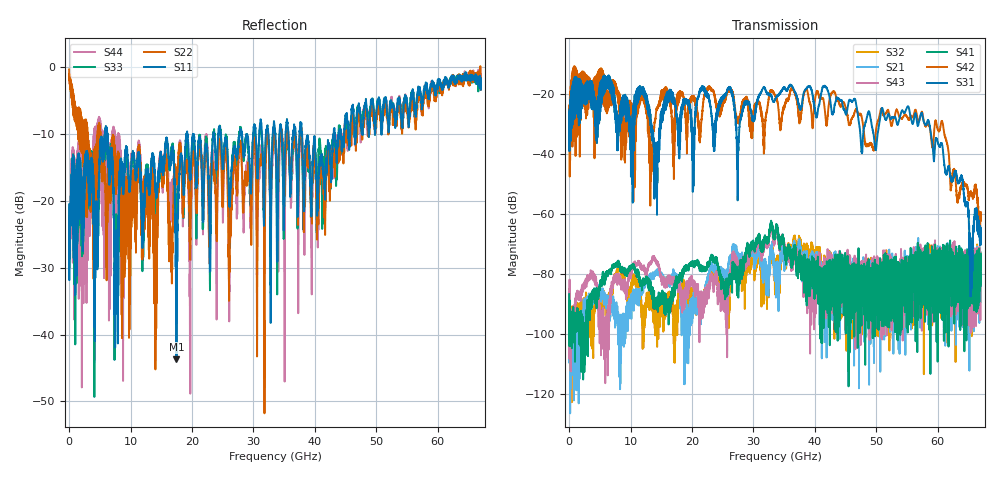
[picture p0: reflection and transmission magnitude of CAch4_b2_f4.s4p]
!Agilent Technologies,N5247A,US51170199,A.09.90.13
!Agilent N5247A: A.09.90.13
!Date: Thursday, October 18, 2018 11:44:51
!Correction: S11(Full 4 Port(1,2,3,4))
!S12(Full 4 Port(1,2,3,4))
!S13(Full 4 Port(1,2,3,4))
!S14(Full 4 Port(1,2,3,4))
!S21(Full 4 Port(1,2,3,4))
!S22(Full 4 Port(1,2,3,4))
!S23(Full 4 Port(1,2,3,4))
!S24(Full 4 Port(1,2,3,4))
!S31(Full 4 Port(1,2,3,4))
!S32(Full 4 Port(1,2,3,4))
!S33(Full 4 Port(1,2,3,4))
!S34(Full 4 Port(1,2,3,4))
!S41(Full 4 Port(1,2,3,4))
!S42(Full 4 Port(1,2,3,4))
!S43(Full 4 Port(1,2,3,4))
!S44(Full 4 Port(1,2,3,4))
!S4P File: Measurements: <S11,S12,S13,S14>,
!<S21,S22,S23,S24>,
!<S31,S32,S33,S34>,
!<S41,S42,S43,S44>:
# Hz S  dB  R 50
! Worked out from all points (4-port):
!   6701 points, 10 MHz to 67 GHz, reference 50 ohm
!   strongest paths, dB at 10 MHz, 16.76 GHz, 33.51 GHz, 50.25 GHz, 67 GHz:
!     S31: -30.8, -22.6, -21.9, -32.7, -65.4
!     S42: -29.6, -28.7, -20.3, -28.8, -59.4
!     S41: -86.7, -85.6, -66.7, -78.8, -83.8
!     S43: -85.9, -82.6, -67.4, -80.2, -76.8
!     S21: -85.4, -80.2, -81.8, -79.9, -77.8
!     S32: -91.4, -88.6, -79.1, -93.8, -72.9
!   lowest |S11| = -43.7 dB at 17.48 GHz (marker M1), VSWR 1.01, Z = 49.3 - j0.0152 ohm
!   |S11| at or under -10 dB: start of sweep to 5.848 GHz; 6.251 GHz to 19.13 GHz (12.88 GHz wide, 101 % of centre); 37.91 GHz to 43.06 GHz (5.145 GHz wide, 12.7 % of centre)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
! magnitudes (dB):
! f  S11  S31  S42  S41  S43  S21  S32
! 10 MHz  -20.5  -30.8  -29.6  -86.7  -85.9  -85.4  -91.4
! 8.809 GHz  -17.0  -20.4  -32.9  -78.7  -83.9  -97.6  -80.6
! 14.19 GHz  -18.7  -40.1  -25.5  -89.4  -76.2  -79.0  -91.5
! 17.48 GHz  -43.7  -27.4  -23.5  -82.2  -82.7  -81.0  -92.9
! 32.92 GHz  -17.8  -20.4  -18.7  -63.4  -64.2  -72.5  -72.9
! 55.1 GHz  -6.3  -24.0  -27.8  -76.6  -86.9  -77.8  -79.3
! 67 GHz  -3.4  -65.4  -59.4  -83.8  -76.8  -77.8  -72.9
